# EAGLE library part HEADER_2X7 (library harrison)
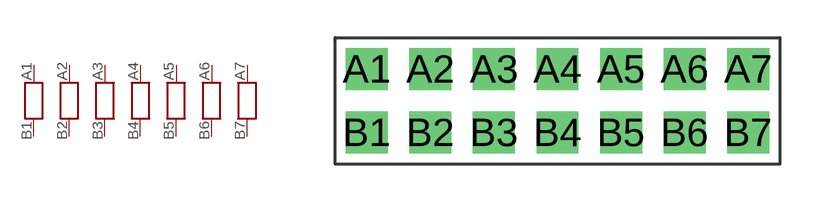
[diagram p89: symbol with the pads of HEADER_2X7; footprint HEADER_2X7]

Designator prefix S

## HEADER_2X7  [HEADER_2X7]
A1  A1  pas
A2  A2  pas
A3  A3  pas
A4  A4  pas
A5  A5  pas
A6  A6  pas
A7  A7  pas
B1  B1  pas
B2  B2  pas
B3  B3  pas
B4  B4  pas
B5  B5  pas
B6  B6  pas
B7  B7  pas

## Footprint HEADER_2X7 (pad centres in mm)
drill 0.813 pad 1.676 square: A1 -7.62,1.27; A2 -5.08,1.27; A3 -2.54,1.27; A4 0,1.27; A5 2.54,1.27; A6 5.08,1.27; A7 7.62,1.27; B1 -7.62,-1.27; B2 -5.08,-1.27; B3 -2.54,-1.27; B4 0,-1.27; B5 2.54,-1.27; B6 5.08,-1.27; B7 7.62,-1.27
